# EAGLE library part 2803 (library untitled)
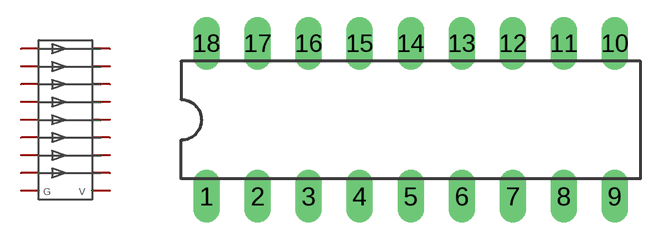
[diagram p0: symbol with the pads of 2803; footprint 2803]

Designator prefix IC

## 2803ULN2803  [2803]
1  P$1  pas
2  P$2  pas
3  P$3  pas
4  P$4  pas
5  P$5  pas
6  P$6  pas
7  P$7  pas
8  P$8  pas
9  P$9  pas
10  P$10  pas
11  P$11  pas
12  P$12  pas
13  P$13  pas
14  P$14  pas
15  P$15  pas
16  P$16  pas
17  P$17  pas
18  P$18  pas

## Footprint 2803 (pad centres in mm)
drill 0.813 long: 1 -10.16,-3.81; 2 -7.62,-3.81; 3 -5.08,-3.81; 4 -2.54,-3.81; 5 0,-3.81; 6 2.54,-3.81; 7 5.08,-3.81; 8 7.62,-3.81; 9 10.16,-3.81; 10 10.16,3.81; 11 7.62,3.81; 12 5.08,3.81; 13 2.54,3.81; 14 0,3.81; 15 -2.54,3.81; 16 -5.08,3.81; 17 -7.62,3.81; 18 -10.16,3.81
